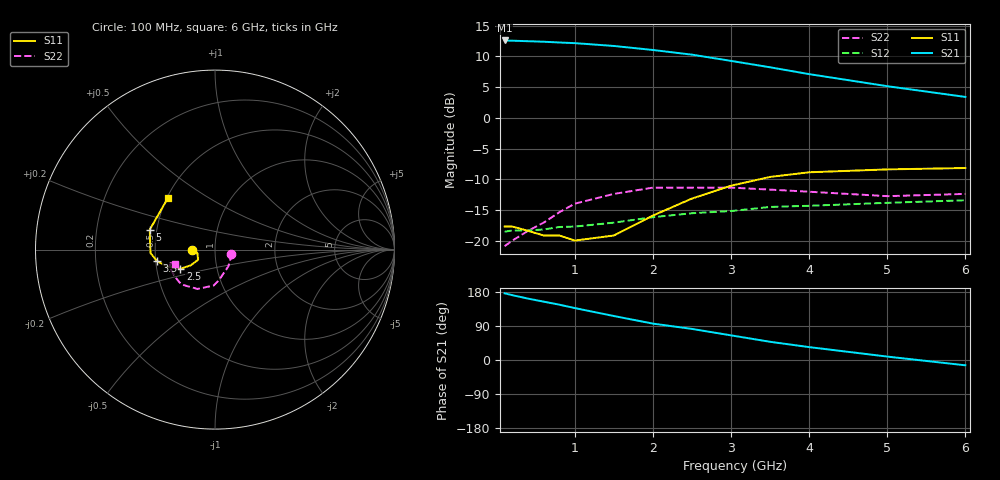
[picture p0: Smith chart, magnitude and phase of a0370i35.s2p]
!  MSA-0370 S AND NOISE PARAMETERS
!  Id=35mA  LAST UPDATED 07-22-92
# ghz s ma r 50
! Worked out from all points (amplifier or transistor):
!   14 points, 100 MHz to 6 GHz, reference 50 ohm
!   highest |S21| = 12.6 dB at 100 MHz (marker M1)
!   |S21| within 3 dB of that: start of sweep to 2.837 GHz
!   unconditionally stable (mu >= 1): start of sweep to end of sweep
!   at 400 MHz: K = 1.20, MAG = 12.7 dB, |S12| = -18.3 dB
!   at 2 GHz: K = 1.05, MAG = 12.2 dB, |S12| = -16.2 dB
!   at 6 GHz: K = 1.33, MAG = 5.0 dB, |S12| = -13.4 dB
!   lowest NFmin = 5.60 dB at 100 MHz
!   S11 on the Smith chart (normalised r, x): 100 MHz: 0.77, -0.00; 2.5 GHz: 0.66, -0.15; 3.5 GHz: 0.51, -0.07; 5 GHz: 0.46, +0.12; 6 GHz: 0.51, +0.35
0.1  0.13 -179.0  4.27 176.0  0.118 2.0  0.09 -14.0
0.2  0.13 -180.0  4.25 171.0  0.121 2.0  0.1 -29.0
0.4  0.12 -180.0  4.21 162.0  0.121 4.0  0.12 -52.0
0.6  0.11 -178.0  4.17 154.0  0.123 6.0  0.14 -70.0
0.8  0.11 -174.0  4.11 146.0  0.129 8.0  0.17 -82.0
1  0.1 -168.0  4.06 137.0  0.13 8.0  0.2 -92.0
1.5  0.11 -149.0  3.85 116.0  0.14 11.0  0.24 -114.0
2  0.16 -147.0  3.57 96.0  0.155 11.0  0.27 -134.0
2.5  0.22 -151.0  3.27 82.0  0.167 14.0  0.27 -146.0
3  0.28 -160.0  2.91 65.0  0.174 11.0  0.27 -159.0
3.5  0.33 -169.0  2.58 48.0  0.188 7.0  0.26 -163.0
4  0.36 -177.0  2.27 34.0  0.192 3.0  0.25 -162.0
5  0.38 163.0  1.81 9.0  0.203 -5.0  0.23 -153.0
6  0.39 132.0  1.48 -14.0  0.213 -13.0  0.24 -160.0
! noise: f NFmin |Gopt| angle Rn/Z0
0.1  5.6  0.04  4  0.83
0.5  5.8  0.05  25  0.83
1  6  0.04  47  0.82
2  6.5  0.05  107  0.79
